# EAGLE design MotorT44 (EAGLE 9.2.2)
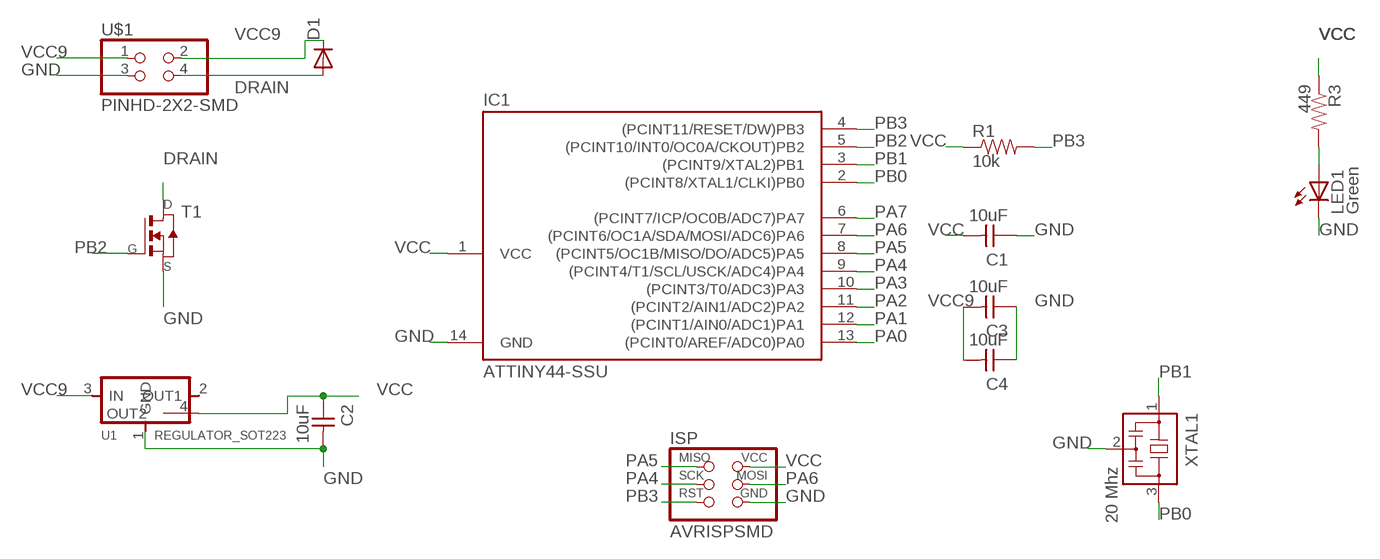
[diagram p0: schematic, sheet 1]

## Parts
C1  10uF  CAP-UNPOLARIZEDFAB  [C1206FAB]
C2  10uF  CAP-UNPOLARIZEDFAB  [C1206FAB]
C3  10uF  CAP-UNPOLARIZEDFAB  [C1206FAB]
C4  10uF  CAP-UNPOLARIZEDFAB  [C1206FAB]
D1  DIODESOD123  [SOD123]
IC1  ATTINY44-SSU  [SOIC14]
ISP  AVRISPSMD  [2X03SMD]
LED1  Green  LEDFAB1206  [LED1206FAB]
R1  10k  RESISTOR1206  [1206]
R3  449  RESISTOR1206  [1206]
T1  NMOSFETTO252  [TO252]
U1  REGULATOR_SOT223  [SOT223]
U$1  PINHD-2X2-SMD  [2X02SMD]
XTAL1  20 Mhz  RESONATOR  [EFOBM]

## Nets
DRAIN: D1.ANODE(A) T1.3(D) U$1.4
GND: C1.1 C2.2 C3.1 C4.1 IC1.14(GND) ISP.6(GND) LED1.2(C) T1.2(S) U1.1(GND) U$1.3 XTAL1.2
N$2: LED1.1(A) R3.2
PA0: IC1.13((PCINT0/AREF/ADC0)PA0)
PA1: IC1.12((PCINT1/AIN0/ADC1)PA1)
PA2: IC1.11((PCINT2/AIN1/ADC2)PA2)
PA3: IC1.10((PCINT3/T0/ADC3)PA3)
PA4: IC1.9((PCINT4/T1/SCL/USCK/ADC4)PA4) ISP.3(SCK)
PA5: IC1.8((PCINT5/OC1B/MISO/DO/ADC5)PA5) ISP.1(MISO)
PA6: IC1.7((PCINT6/OC1A/SDA/MOSI/ADC6)PA6) ISP.4(MOSI)
PA7: IC1.6((PCINT7/ICP/OC0B/ADC7)PA7)
PB0: IC1.2((PCINT8/XTAL1/CLKI)PB0) XTAL1.3
PB1: IC1.3((PCINT9/XTAL2)PB1) XTAL1.1
PB2: IC1.5((PCINT10/INT0/OC0A/CKOUT)PB2) T1.1(G)
PB3: IC1.4((PCINT11/RESET/DW)PB3) ISP.5(RST) R1.2
VCC: C1.2 C2.1 IC1.1(VCC) ISP.2(VCC) R1.1 R3.1 U1.4(OUT2)
VCC9: C3.2 C4.2 D1.CATHODE(C) U1.3(IN) U$1.1 U$1.2
Unconnected: U1.2(OUT1)

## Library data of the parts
C1-C4 = fab:CAP-UNPOLARIZED
D1 = fab:DIODE: DIODE
IC1 = fab:ATTINY44
ISP = fab:AVRISP
LED1 = fab:LED: LED
R1 R3 = SparkFun-Resistors:RESISTOR: Generic Resistor Package
T1 = fab:NMOSFET: MOS FET
U1 = fab:REGULATOR_SOT223
U$1 = fab:PINHD-2X2-SMD
XTAL1 = fab:RESONATOR

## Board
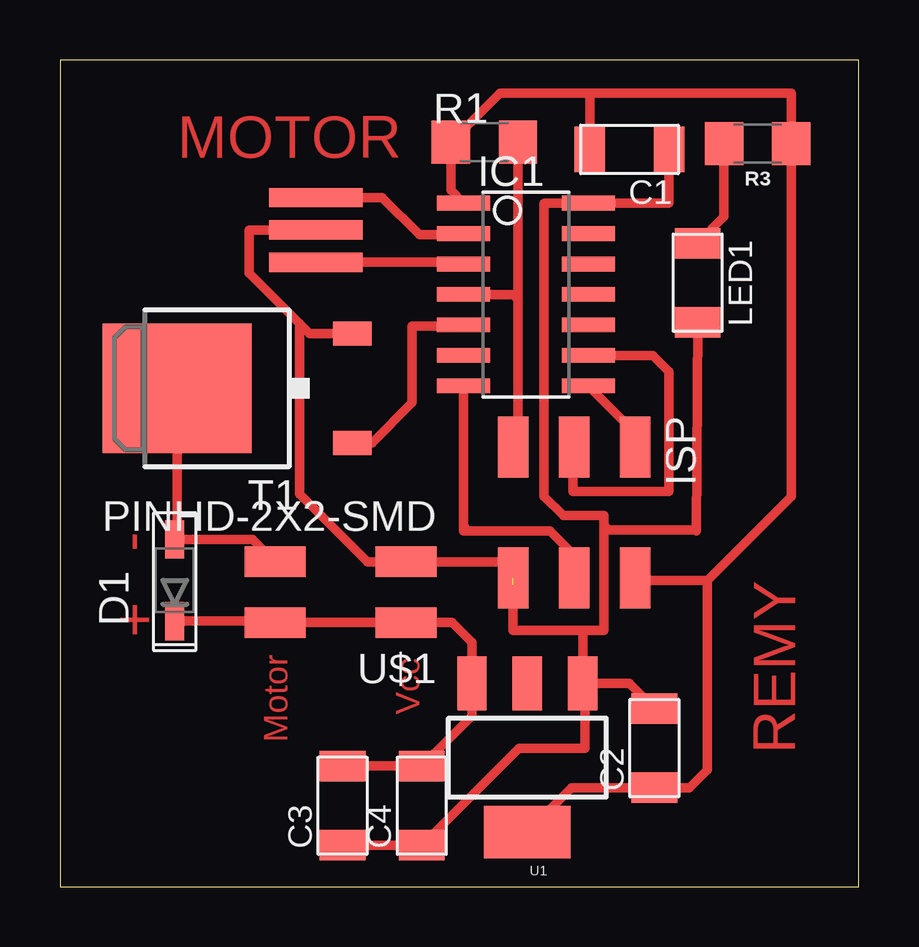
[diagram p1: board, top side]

Size 33.3 x 34.46 mm. Coordinates in mm from the lower left corner, seen from the top.
Outline: 0,0 33.3,0 33.3,34.46 0,34.46 0,0
Copper layers (1*16): Top 0.035mm / dielectric 1.5mm / Bottom 0.035mm
Design rules "default *": minimum track width 0.4mm, minimum drill 0.4mm, track to track 0.3mm, track to pad 0.3mm, pad to pad 0.3mm, via to via 6mil, smd to smd 0.3mm, copper to edge 40mil, drill to drill 6mil, minimum pad ring 10mil, minimum via ring 8mil, stop-mask expansion 4mil, vias tented up to drill 0mil, thermal gap 10mil

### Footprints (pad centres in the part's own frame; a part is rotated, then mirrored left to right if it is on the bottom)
C1206FAB = smd 1.27 x 1.905: 1 -1.651,0; 2 1.651,0
SOD123 = smd 1.6 x 0.8: ANODE 1.7,0; CATHODE -1.7,0
SOIC14 = smd 0.61 x 2.21: 1 -3.81,-2.603; 2 -2.54,-2.603; 3 -1.27,-2.603; 4 0,-2.603; 5 1.27,-2.603; 6 2.54,-2.603; 7 3.81,-2.603; 8 3.81,2.603; 9 2.54,2.603; 10 1.27,2.603; 11 0,2.603; 12 -1.27,2.603; 13 -2.54,2.603; 14 -3.81,2.603
2X03SMD = smd 2.54 x 1.27: 1 -2.54,2.54; 2 2.92,2.54; 3 -2.54,0; 4 2.92,0; 5 -2.54,-2.54; 6 2.92,-2.54
LED1206FAB = smd 1.27 x 1.905: 1 -1.651,0; 2 1.651,0
1206 = smd 1.6 x 1.8: 1 -1.4,0; 2 1.4,0
TO252 = smd 1 x 1.6: 1 -2.28,-4.8; 2 2.28,-4.8 | smd 5.4 x 6.2: 3 0,2.5
SOT223 = smd 1.219 x 2.235: 1 -2.311,-3.099; 2 0,-3.099; 3 2.311,-3.099 | smd 3.6 x 2.2: 4 0,3.099
2X02SMD = smd 2.54 x 1.27: 1 -2.54,1.27; 2 2.92,1.27; 3 -2.54,-1.27; 4 2.92,-1.27
EFOBM = smd 0.8 x 3.9: 1 -1.35,0; 2 0,0; 3 1.35,0

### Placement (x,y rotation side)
C1  23.74,30.73 180 top
C2  24.78,5.77 90 top
C3  11.78,3.37 90 top
C4  15.08,3.37 90 top
D1  4.78,12.77 90 top
IC1  19.43,24.68 270 top
ISP  21.43,15.79 270 top
LED1  26.58,25.17 270 top
R1  17.69,31.03 0 top
R3  29.08,30.97 180 top
T1  7.38,20.77 90 top
U1  19.48,5.37 180 top
U$1  11.88,12.27 180 top
XTAL1  10.67,27.38 90 top

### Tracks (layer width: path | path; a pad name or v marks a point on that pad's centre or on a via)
DRAIN
  Top 0.4: T1.3 4.88,14.57 D1.ANODE 8.03,14.47 U$1.4
GND  (1 unrouted)
  Top 0.4: 18.76,13.01 ISP.6 | 25.59,30.93 C1.1 25.39,28.49 IC1.14 | 21.92,28.37 IC1.14 | 18.88,12.57 18.89,12.57 | 21.78,10.67 18.88,10.67 18.89,10.68 18.89,12.57 | 21.78,10.67 22.68,10.67 22.68,15.07 | IC1.14 20.2,28.49 20.18,28.47 20.18,16.27 20.98,15.47 22.68,15.47 22.68,15.07 | XTAL1.2 10.57,27.27 10.47,27.37 7.88,27.37 7.88,25.57 9.98,23.47 | 22.68,15.07 22.88,14.87 26.48,14.87 26.53,14.82 LED1.2 | T1.2 10.4,23.05 9.98,23.47 | 18.89,12.57 18.89,13.38 18.98,13.47 18.91,13.54 U$1.3 12.81,13.54 9.98,16.37 9.98,23.47 | U1.1 21.79,10.66 21.78,10.67 | U1.1 23.74,8.47 C2.2 | 10.98,1.37 11.33,1.72 C3.1 C4.1 19.13,5.77 21.88,5.77 21.88,8.38 U1.1
N$2
  Top 0.4: LED1.1 27.68,27.92 R3.2
PA1
  Top 0.4: IC1.12 22.06,25.97
PA4
  Top 0.152: ISP.3
  Top 0.4: ISP.3 21.38,18.29 21.38,16.47 25.38,16.47 25.38,21.47 24.71,22.14 IC1.9
PA5
  Top 0.4: ISP.1 23.97,18.94 IC1.8
PA6
  Top 0.4: IC1.7 16.83,15.03 | 16.83,15.03 16.83,14.83 20.43,14.83 21.43,13.82 ISP.4 | 16.83,15.03 16.88,14.97
PA7
  Top 0.4: 16.8,22.17 IC1.6
PB0
  Top 0.4: XTAL1.3 10.98,28.73 | 10.98,28.73 13.43,28.73 14.98,27.17 16.78,27.17 IC1.2 | 10.93,28.67 10.98,28.73
PB1
  Top 0.4: XTAL1.1 16.76,26.03 IC1.3
PB2
  Top 0.4: 16.8,23.44 IC1.5 16.79,23.37 14.68,23.37 14.68,20.17 13,18.49 T1.1
PB3
  Top 0.4: ISP.5 19.09,18.54 19.09,24.47 | 16.94,24.57 IC1.4 18.88,24.68 19.09,24.47 | R1.2 19.09,24.47
VCC
  Top 0.4: R1.1 16.29,29.03 IC1.1 | R1.1 18.33,33.07 22.09,33.07 | C1.2 22.09,33.07 | 16.23,30.97 R1.1 | 22.09,33.07 30.48,33.07 R3.1 30.48,16.27 26.98,12.77 | 23.88,12.79 ISP.2 24.07,12.77 26.98,12.77 | 26.98,12.77 26.98,4.87 26.23,4.12 C2.1 21.33,4.12 U1.4
VCC9
  Top 0.4: D1.CATHODE 8.89,11.07 U$1.2 U$1.1 16.35,11 17.18,10.17 17.17,10.16 U1.3 17.17,7.11 C4.2 C3.2

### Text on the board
Top: MOTOR | - | REMY | + | Motor | Vcc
